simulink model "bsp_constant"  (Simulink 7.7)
settings: Solver=ode45  StartTime=0.0  StopTime=10.0  RelTol=1e-3

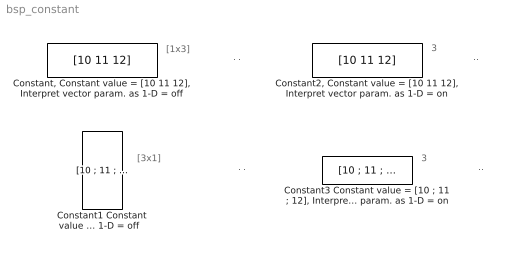
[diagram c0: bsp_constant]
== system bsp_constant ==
  note: ...
  note: ...
  note: ...
  note: ...
  note: [1x3]
  note: [3x1]
  note: 3
  note: 3
  "Constant, Constant value = [10 11 12], Interpret vector param. as 1-D = off" : Constant  Value=[10 11 12]  VectorParams1D=off
  "Constant1 Constant value = [10 ; 11 ; 12], Interpret vector param. as 1-D = off  " : Constant  Value=[10 ; 11 ; 12]  VectorParams1D=off
  "Constant2, Constant value = [10 11 12], Interpret vector param. as 1-D = on" : Constant  Value=[10 11 12]
  "Constant3 Constant value = [10 ; 11 ; 12], Interpret vector param. as 1-D = on" : Constant  Value=[10 ; 11 ; 12]
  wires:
  "Constant, Constant value = [10 11 12], Interpret vector param. as 1-D = off"/1 -> ?
  "Constant1 Constant value = [10 ; 11 ; 12], Interpret vector param. as 1-D = off  "/1 -> ?
  "Constant2, Constant value = [10 11 12], Interpret vector param. as 1-D = on"/1 -> ?
  "Constant3 Constant value = [10 ; 11 ; 12], Interpret vector param. as 1-D = on"/1 -> ?
